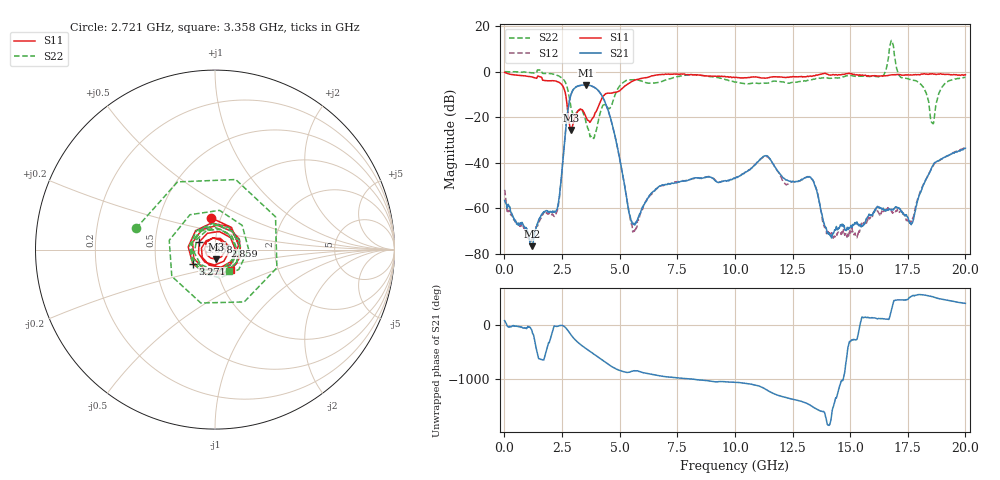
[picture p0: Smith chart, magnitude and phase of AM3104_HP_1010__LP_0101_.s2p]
!Created with skrf (http://scikit-rf.org).
# Hz S RI R 50.0
!freq ReS11 ImS11 ReS21 ImS21 ReS12 ImS12 ReS22 ImS22
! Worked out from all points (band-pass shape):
!   1601 points, 10 MHz to 20 GHz, reference 50 ohm
!   highest |S21| = -5.83 dB at 3.558 GHz (marker M1); lowest = -76.6 dB at 1.197 GHz (marker M2)
!   |S21| within 3 dB of the highest: 2.938 GHz to 4.118 GHz (1.18 GHz wide, 33.5 % of centre)
!   lowest |S11| = -25.6 dB at 2.896 GHz (marker M3), VSWR 1.11, Z = 50.5 - j5.27 ohm
!   |S11| at or under -10 dB: 2.656 GHz to 4.357 GHz (1.7 GHz wide, 48.5 % of centre)
!   |S22| runs from -29.5 to 13.6 dB; largest |S21 - S12| = 0.025
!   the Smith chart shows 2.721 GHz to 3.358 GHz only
!   S11 on the Smith chart (normalised r, x): 2.721 GHz: 0.90, +0.33; 2.859 GHz: 1.11, +0.05; 3.058 GHz: 0.84, +0.07; 3.271 GHz: 0.77, -0.12; 3.358 GHz: 1.16, -0.27
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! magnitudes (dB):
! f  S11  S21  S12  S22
! 10 MHz  -0.4  -56.5  -51.9  -0.1
! 1.197 GHz  -2.3  -76.6  -73.8  -0.6
! 2.271 GHz  -4.3  -60.7  -61.6  -1.6
! 2.721 GHz  -14.9  -19.7  -19.7  -6.8
! 2.859 GHz  -24.8  -11.2  -11.3  -13.9
! 2.896 GHz  -25.6  -9.9  -10.0  -15.9
! 3.058 GHz  -20.2  -7.2  -7.2  -18.7
! 3.271 GHz  -16.7  -6.1  -6.2  -17.0
! 3.346 GHz  -16.6  -6.0  -6.0  -16.8
! 3.358 GHz  -16.7  -6.0  -6.0  -16.8
! 3.558 GHz  -20.3  -5.8  -5.9  -22.8
! 4.52 GHz  -9.5  -17.6  -17.7  -16.2
! 5.595 GHz  -4.1  -66.8  -70.0  -3.6
! 6.682 GHz  -1.4  -50.7  -50.6  -4.8
! 10.01 GHz  -2.7  -46.9  -46.8  -4.6
! 11.33 GHz  -2.9  -37.0  -37.4  -5.1
! 13.34 GHz  -2.1  -47.1  -47.2  -3.6
! 14.12 GHz  -1.5  -71.7  -70.9  -2.9
! 16.68 GHz  -1.6  -60.4  -60.5  7.2
! 17.66 GHz  -1.5  -66.6  -65.9  -3.8
! 18.56 GHz  -0.9  -41.6  -41.8  -22.6
! 20 GHz  -1.4  -33.6  -33.2  -2.5
